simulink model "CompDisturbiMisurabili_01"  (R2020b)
settings: Solver=FixedStepAuto  StartTime=0.0  StopTime=50  FixedStep=0.001  RelTol=1e-3  EnableMultiTasking=on
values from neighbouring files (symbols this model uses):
  tau = 0.005    [AnticipoSetpoint2020_script.m]    (also in CompDisturbiMisurabili_01_script.m = 0.01)

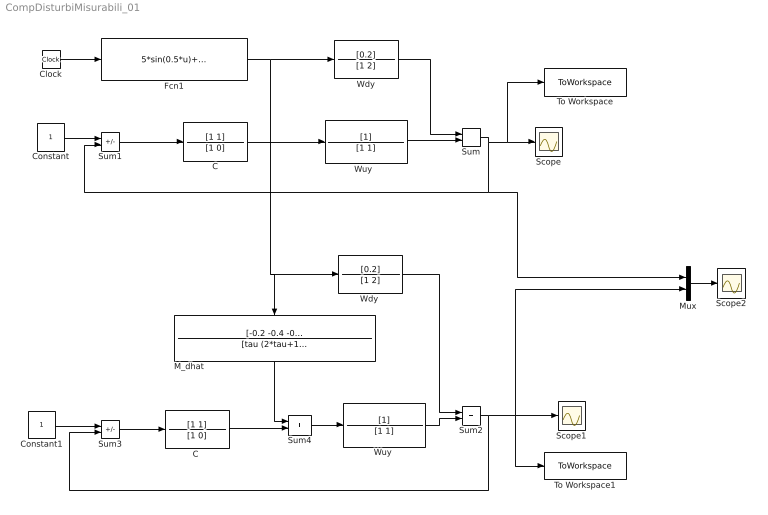
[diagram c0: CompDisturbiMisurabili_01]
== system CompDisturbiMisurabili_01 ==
  C : TransferFcn  Numerator=[1 1]  Denominator=[1 0]
  "C " : TransferFcn  Numerator=[1 1]  Denominator=[1 0]
  Clock : Clock
  Constant : Constant
  Constant1 : Constant
  Fcn1 : Fcn  Expr=5*sin(0.5*u)+cos(u)
  "M_dhat " : TransferFcn  Numerator=[-0.2 -0.4 -0.2]  Denominator=[tau (2*tau+1) 2]
  Mux : Mux  Inputs=2
  Scope : Scope
  Scope1 : Scope
  Scope2 : Scope
  Sum : Sum
  Sum1 : Sum  Inputs=+-
  Sum2 : Sum
  Sum3 : Sum  Inputs=+-
  Sum4 : Sum
  To Workspace : ToWorkspace  VariableName=y  SaveFormat=Timeseries  SampleTime=-1
  To Workspace1 : ToWorkspace  VariableName=y_comp  SaveFormat=Timeseries  SampleTime=-1
  Wdy : TransferFcn  Numerator=[0.2]  Denominator=[1 2]
  "Wdy " : TransferFcn  Numerator=[0.2]  Denominator=[1 2]
  "Wuy " : TransferFcn
  "Wuy  " : TransferFcn
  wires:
  C/1 -> "Wuy  "/1
  Sum1/1 -> C/1
  Sum/1 -> To Workspace/1, Scope/1, Mux/1, Sum1/2
  "Wuy "/1 -> Sum2/2
  Sum3/1 -> "C "/1
  Sum2/1 -> Mux/2, To Workspace1/1, Scope1/1, Sum3/2
  Constant/1 -> Sum1/1
  "Wdy "/1 -> Sum2/1
  "C "/1 -> Sum4/2
  Sum4/1 -> "Wuy "/1
  "M_dhat "/1 -> Sum4/1
  Mux/1 -> Scope2/1
  Wdy/1 -> Sum/1
  "Wuy  "/1 -> Sum/2
  Constant1/1 -> Sum3/1
  Fcn1/1 -> Wdy/1, "Wdy "/1, "M_dhat "/1
  Clock/1 -> Fcn1/1
